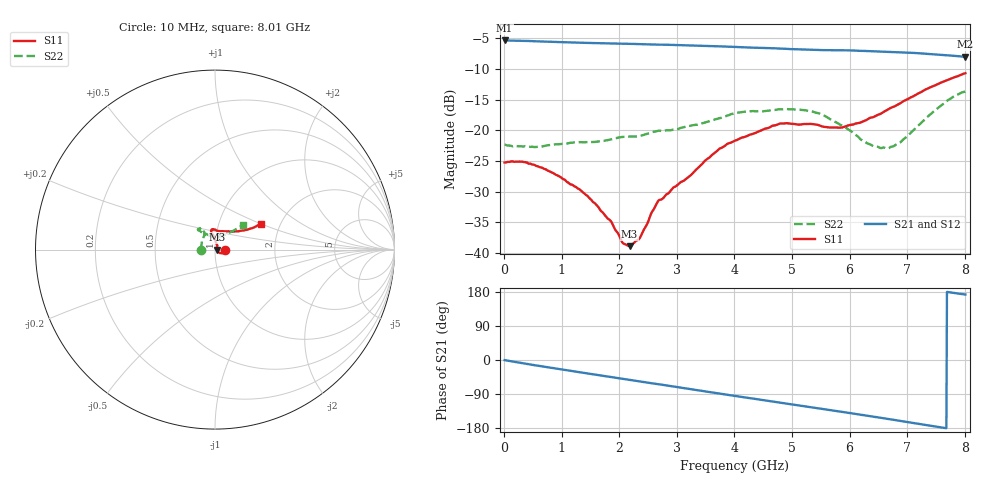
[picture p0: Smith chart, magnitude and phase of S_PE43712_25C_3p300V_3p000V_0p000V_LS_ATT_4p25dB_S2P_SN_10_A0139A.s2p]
! DEVICE ID: PE43712
! File Path: z:\PE43713\PE43713_CHAR_NOM_04292014\AMB\3p300\LS_ATT_4p25dB\PE43713_AMB_3p300V_3p000V_0p000V_LS_ATT_4p25dB_S2P_SN_10_A0139A.s2p
! Serial: 10
! Lot: A0139A
! Temp: 25C
! VDD: 3.300
! VSS: 0.000
! Control_Hi: 3.000
! Control_Lo: 0.000
! Attenuation Step: 4.25dB
! Port 1: RF1
! Port 2: RF2
! ThroughPath:1-2
! IDD: 0.0001468835
! ISS: -1.071e-007
#  Hz  S  RI  R  50
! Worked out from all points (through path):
!   801 points, 10 MHz to 8.01 GHz, reference 50 ohm
!   highest |S21| = -5.35 dB at 10 MHz (marker M1); lowest = -8.0 dB at 8.01 GHz (marker M2)
!   group delay of S21, straight-line fit = 64.3 ps
!   lowest |S11| = -38.9 dB at 2.18 GHz (marker M3), VSWR 1.02, Z = 51.1 + j0.0286 ohm
!   |S11| at or under -10 dB: start of sweep to end of sweep
!   |S22| runs from -23.0 to -13.7 dB; largest |S21 - S12| = 0.0016
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1e7  0.0547 -0.000162  0.5401 -0.00313  0.5398 -0.00277  -0.0763 0.000357
3.4e8  0.054 -0.0113  0.5285 -0.083  0.5282 -0.0818  -0.0737 0.0045
6.3e8  0.0469 -0.0172  0.5094 -0.1473  0.5093 -0.1473  -0.0731 0.00921
9.6e8  0.0369 -0.02  0.4783 -0.2141  0.4784 -0.2141  -0.0756 0.0156
1.35e9  0.0256 -0.0187  0.4331 -0.2831  0.433 -0.2831  -0.0763 0.0243
1.85e9  0.0162 -0.00857  0.3628 -0.3593  0.3629 -0.3592  -0.0733 0.0413
2.07e9  0.0116 -0.00302  0.3277 -0.3882  0.3278 -0.388  -0.0738 0.0486
2.18e9  0.0114 0.00028  0.3094 -0.4014  0.3095 -0.4012  -0.0721 0.0521
2.36e9  0.0107 0.00793  0.2775 -0.4211  0.2775 -0.4209  -0.0672 0.0601
2.68e9  0.0128 0.0234  0.2196 -0.4482  0.2197 -0.4482  -0.0586 0.0801
2.99e9  0.00788 0.0343  0.1602 -0.4694  0.1602 -0.4696  -0.0583 0.0832
3.24e9  0.00352 0.0428  0.1105 -0.4791  0.1107 -0.4792  -0.0596 0.0913
3.71e9  -0.00199 0.0687  0.0183 -0.483  0.0181 -0.4831  -0.0651 0.1059
4.01e9  -0.00974 0.0818  -0.04 -0.4769  -0.04 -0.4769  -0.0771 0.1143
4.79e9  -0.0186 0.1119  -0.1776 -0.4283  -0.1776 -0.4285  -0.0938 0.1151
5.35e9  -0.00402 0.1122  -0.2597 -0.3717  -0.2595 -0.3714  -0.0931 0.1078
5.87e9  0.0269 0.1019  -0.3275 -0.3082  -0.3268 -0.3083  -0.06 0.0914
6.33e9  0.0719 0.1019  -0.3734 -0.2377  -0.3725 -0.2374  -0.021 0.0747
6.68e9  0.1094 0.1013  -0.3977 -0.1778  -0.3973 -0.1778  0.0119 0.0705
6.9e9  0.1341 0.1023  -0.4089 -0.1389  -0.4085 -0.1389  0.0337 0.0741
7.7e9  0.224 0.1274  -0.4086 0.00355  -0.4082 0.00318  0.1279 0.1198
8.01e9  0.2547 0.1427  -0.3942 0.0504  -0.3935 0.0497  0.1552 0.1375
